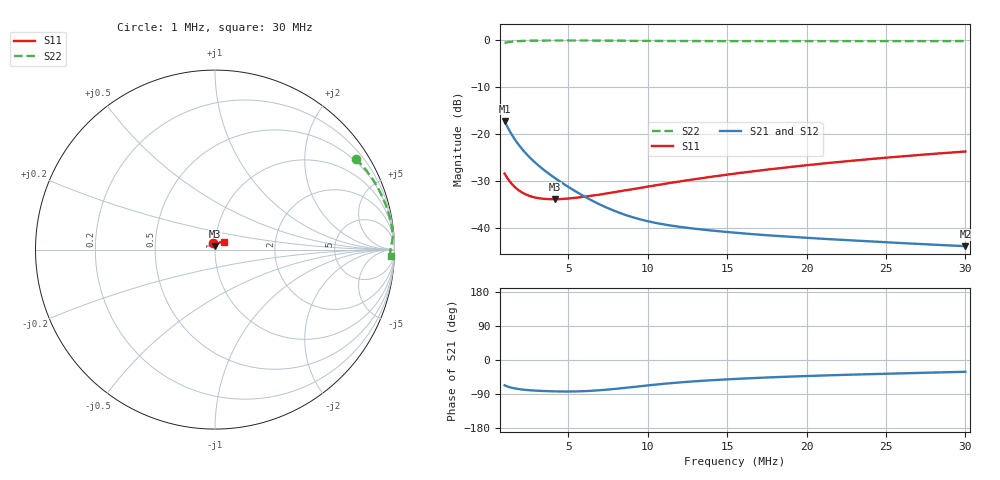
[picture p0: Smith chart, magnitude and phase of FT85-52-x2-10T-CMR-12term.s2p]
! ListType=Log
!!FT85-52 x2 10T CMR 12-term
# MHZ S RI R 50
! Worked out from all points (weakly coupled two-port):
!   101 points, 1 MHz to 30 MHz, reference 50 ohm
!   highest |S21| = -17.21 dB at 1 MHz (marker M1); lowest = -43.8 dB at 30 MHz (marker M2)
!   lowest |S11| = -33.9 dB at 4.172 MHz (marker M3), VSWR 1.04, Z = 50.1 + j2.03 ohm
!   |S11| at or under -10 dB: start of sweep to end of sweep
!   |S22| runs from -0.6 to -0.1 dB; largest |S21 - S12| = 0.00025
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1  -0.0138 0.0354  0.0544 -0.1266  0.0545 -0.1268  0.7837 0.5074
1.185376  -0.0102 0.0322  0.0408 -0.1116  0.0409 -0.1118  0.8384 0.4467
1.312713  -0.00842 0.0304  0.0341 -0.1029  0.0342 -0.1031  0.8651 0.4113
1.453729  -0.00686 0.0287  0.0285 -0.0945  0.0286 -0.0947  0.8877 0.3773
1.782833  -0.00433 0.0258  0.0198 -0.079  0.0198 -0.0791  0.9228 0.3144
2.186442  -0.00242 0.0234  0.0136 -0.0654  0.0137 -0.0655  0.9474 0.2589
2.591755  -0.00107 0.0219  0.00999 -0.0554  0.01 -0.0556  0.9619 0.2183
2.969469  -0.000176 0.0211  0.0078 -0.0484  0.00782 -0.0485  0.9707 0.1894
3.641716  0.00108 0.0204  0.0054 -0.0392  0.00541 -0.0393  0.9802 0.1512
4.172448  0.00191 0.0202  0.00427 -0.0338  0.00428 -0.0339  0.9846 0.1287
5.117033  0.00321 0.0204  0.0032 -0.0266  0.0032 -0.0266  0.9888 0.0982
5.862773  0.00407 0.021  0.00294 -0.0223  0.00294 -0.0224  0.9897 0.0799
6.492571  0.00473 0.0216  0.00301 -0.0194  0.00299 -0.0195  0.9894 0.0674
7.190024  0.00548 0.0224  0.00326 -0.0169  0.00324 -0.017  0.9883 0.0562
8.237875  0.00667 0.0237  0.00375 -0.014  0.00373 -0.0141  0.9862 0.0431
9.438436  0.00803 0.0254  0.00435 -0.0117  0.00433 -0.0118  0.9838 0.032
10.81396  0.00978 0.0274  0.00493 -0.00995  0.00491 -0.01  0.9813 0.0227
12.81861  0.0127 0.0303  0.00545 -0.00829  0.00543 -0.00834  0.9791 0.013
15.72057  0.0174 0.0343  0.00575 -0.00676  0.00574 -0.0068  0.9778 0.00238
20.63659  0.0266 0.0398  0.00582 -0.00514  0.00581 -0.0052  0.9774 -0.0118
25.30843  0.0367 0.0432  0.00569 -0.00413  0.00568 -0.0042  0.9777 -0.0232
30  0.0477 0.0446  0.0055 -0.00332  0.00548 -0.00339  0.9783 -0.0336
